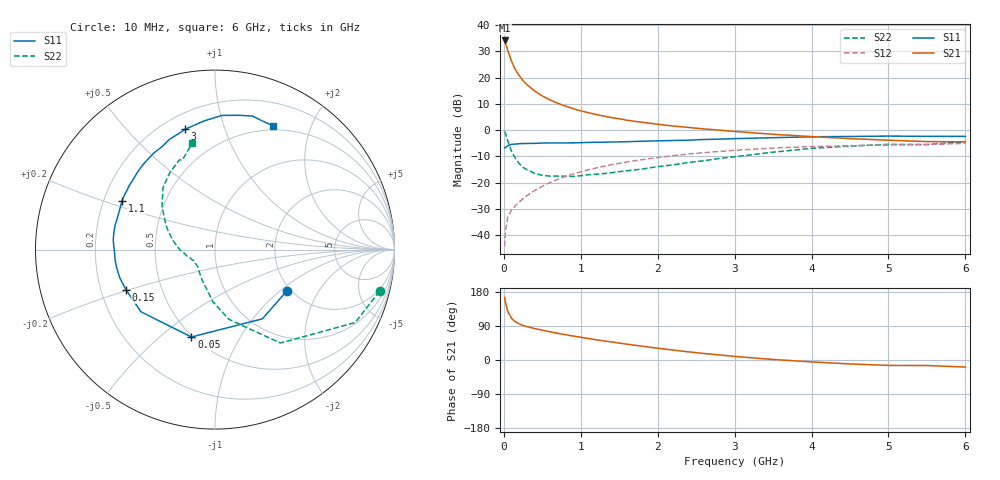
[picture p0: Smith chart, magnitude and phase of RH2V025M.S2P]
! SIEMENS Small Signal Semiconductors
! BFR106
! Si NPN RF Bipolar Junction Transistor in SOT23
! VCE = 2 V  IC = 25 mA
! Common Emitter S-Parameters:  August  1996
# GHz  S  MA  R  50
!  f  S11  S21  S12  S22
! GHz  MAG  ANG  MAG  ANG  MAG  ANG  MAG  ANG
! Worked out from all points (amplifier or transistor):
!   36 points, 10 MHz to 6 GHz, reference 50 ohm
!   highest |S21| = 34.2 dB at 10 MHz (marker M1)
!   |S21| within 3 dB of that: start of sweep to 43.3 MHz
!   unconditionally stable (mu >= 1): 319.4 MHz to 2.527 GHz; 5.11 GHz to end of sweep
!   at 250 MHz: K = 0.94, MSG = 22.5 dB, |S12| = -26.1 dB
!   at 1.4 GHz: K = 1.07, MAG = 7.3 dB, |S12| = -13.1 dB
!   at 6 GHz: K = 1.01, MAG = -0.4 dB, |S12| = -5.0 dB
!   S11 on the Smith chart (normalised r, x): 10 MHz: 1.92, -1.11; 50 MHz: 0.49, -0.64; 150 MHz: 0.31, -0.20; 1.1 GHz: 0.28, +0.23; 3 GHz: 0.29, +0.74; 6 GHz: 0.45, +1.48
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0.01  0.4623 -29.6  51.05 165.5  0.0062 79.5  0.9455 -14.2
0.02  0.4674 -55.6  47.05 153.7  0.0116 71.0  0.8804 -27.5
0.05  0.5043 -105.1  33.5 128.7  0.0219 55.9  0.6355 -55.0
0.1  0.5386 -140.0  20.43 110.0  0.0301 52.3  0.3962 -78.7
0.15  0.544 -155.6  14.22 100.7  0.0365 54.5  0.2905 -92.4
0.2  0.5535 -163.5  10.94 95.3  0.0427 57.9  0.2312 -100.6
0.25  0.5571 -169.7  8.772 91.1  0.0497 59.8  0.1954 -109.3
0.3  0.5593 -173.4  7.361 88.2  0.0566 62.3  0.1773 -115.1
0.4  0.5613 180.0  5.587 83.1  0.0711 64.5  0.1516 -125.3
0.5  0.5695 174.8  4.492 78.6  0.0856 65.9  0.1379 -132.9
0.6  0.5719 170.1  3.77 74.4  0.101 65.9  0.1339 -138.0
0.7  0.5729 166.0  3.257 70.4  0.116 65.9  0.1337 -143.1
0.9  0.5734 159.2  2.573 63.3  0.1468 64.2  0.1315 -151.7
1.1  0.5852 152.5  2.15 56.6  0.1766 62.2  0.142 -157.4
1.3  0.5909 146.1  1.851 50.4  0.2057 59.5  0.1491 -163.5
1.6  0.6041 137.6  1.549 41.7  0.2481 55.3  0.1688 -171.3
2.2  0.6372 122.1  1.201 26.2  0.3271 46.0  0.2187 172.8
3  0.6907 104.0  0.947 9.4  0.414 33.1  0.3119 152.0
3.5  0.7196 94.8  0.836 1.4  0.4571 25.4  0.3816 140.7
4.5  0.7593 80.3  0.692 -10.4  0.5067 10.7  0.4985 120.2
5.5  0.763 69.1  0.607 -14.5  0.5346 1.6  0.5319 109.9
6  0.7623 64.9  0.602 -18.7  0.561 -5.3  0.6074 102.0
